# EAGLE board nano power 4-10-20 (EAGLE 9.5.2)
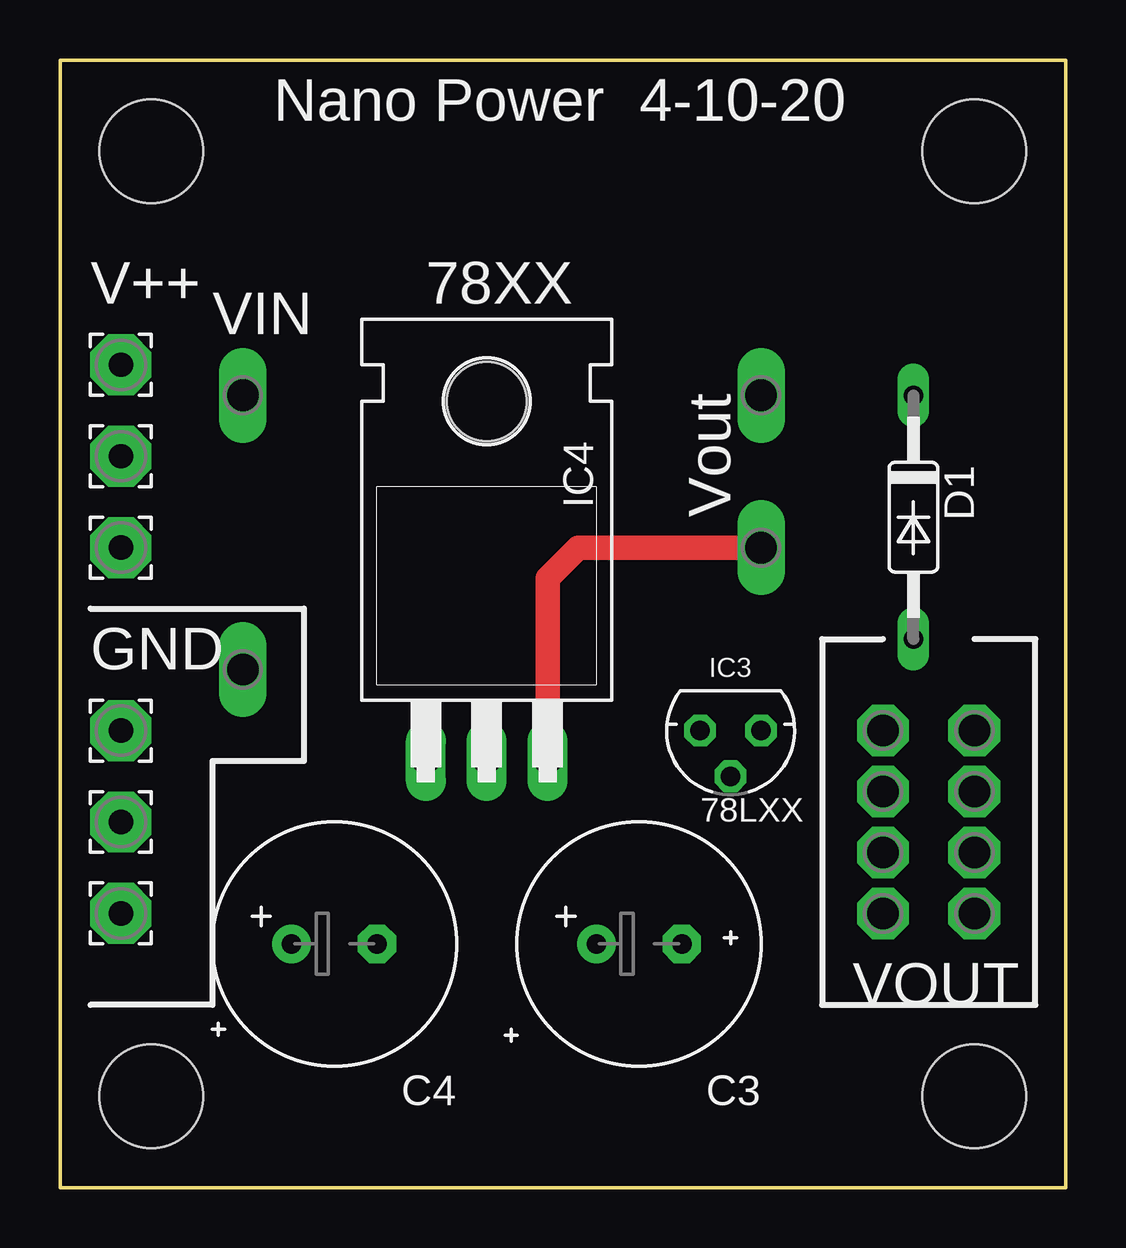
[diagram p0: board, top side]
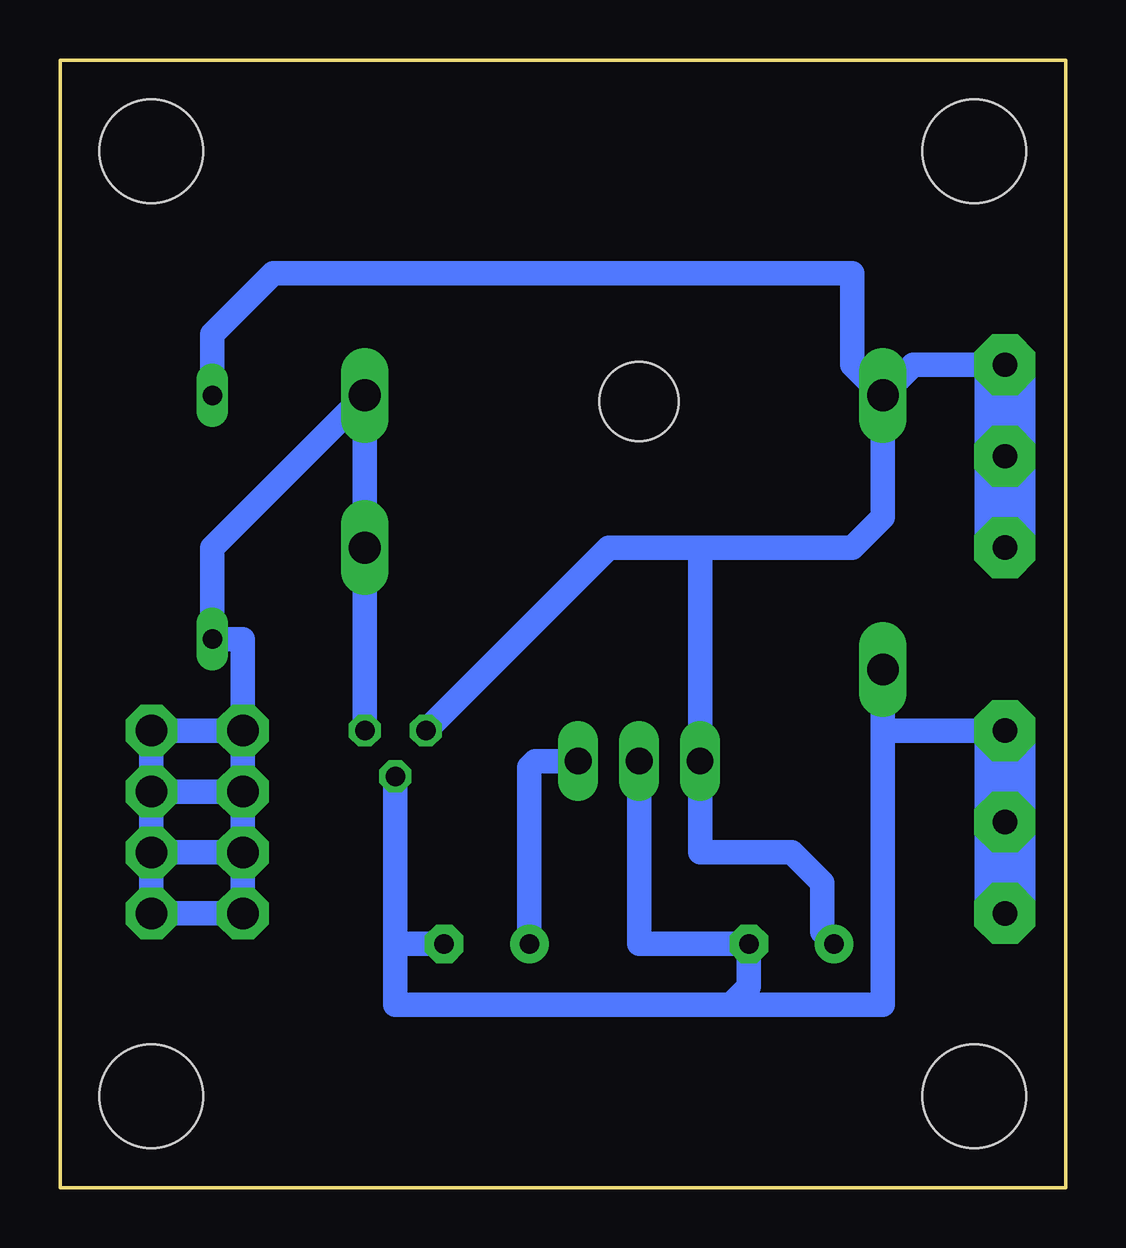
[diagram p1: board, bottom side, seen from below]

Size 41.91 x 46.99 mm. Coordinates in mm from the lower left corner, seen from the top.
Outline: 0,46.99 0,0 41.91,0 41.91,46.99 0,46.99
Copper layers (1*16): Top 0.035mm / dielectric 1.5mm / Bottom 0.035mm
Design rules "default": minimum track width 6mil, minimum drill 0.35mm, track to track 6mil, track to pad 6mil, pad to pad 6mil, via to via 6mil, smd to smd 6mil, copper to edge 40mil, drill to drill 6mil, minimum pad ring 10mil, minimum via ring 8mil, stop-mask expansion 4mil, vias tented up to drill 0mil, thermal gap 10mil
Holes 4.32 mm at 3.81,43.18 38.1,43.18 38.1,3.81 3.81,3.81

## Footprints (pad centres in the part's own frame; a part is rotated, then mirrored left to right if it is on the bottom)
2,54/1,0 = drill 1.016 pad 2.54 octagon: 1 0,0
E3,5-10 = drill 0.813 pad 1.6: + -1.778,0 | drill 0.813 pad 1.6 octagon: - 1.778,0
DO35-10 = drill 0.813 long: A 5.08,0; C -5.08,0
TO220H = drill 1.118 long: 1 -2.54,-10.16; 2 0,-10.16; 3 2.54,-10.16 | hole 3.302: 0,4.826
78LXX = drill 0.813 octagon: GND 0,1.905; IN 1.27,0; OUT -1.27,0
P1-13 = drill 1.321 pad 2.159 octagon: TP 0,0
P1-13Y = drill 1.321 pad 1.905 long: TP 0,0

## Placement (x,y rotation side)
.GND2  [2,54/1,0]  2.54,15.24 0 top
.V++1  [2,54/1,0]  2.54,30.48 0 top
C3  10uF  [E3,5-10]  24.13,10.16 0 top
C4  47uF  [E3,5-10]  11.43,10.16 0 top
D1  1N5404  [DO35-10]  35.56,27.94 270 top
GND1  [2,54/1,0]  2.54,19.05 0 top
GND.2  [2,54/1,0]  2.54,11.43 0 top
IC3  7808T  [TO220H]  17.78,27.94 0 top
IC4  [78LXX]  27.94,19.05 180 top
TP1  TPPAD1-13  [P1-13]  34.29,19.05 0 top
TP2  TPPAD1-13  [P1-13]  34.29,16.51 180 top
TP3  TPPAD1-13  [P1-13]  34.29,13.97 0 top
TP4  TPPAD1-13  [P1-13]  34.29,11.43 0 top
TP13  TPPAD1-13  [P1-13]  38.1,19.05 0 top
TP14  TPPAD1-13  [P1-13]  38.1,16.51 180 top
TP15  TPPAD1-13  [P1-13]  38.1,13.97 0 top
TP16  TPPAD1-13  [P1-13]  38.1,11.43 0 top
V++2  PTR1PAD1-13Y  [P1-13Y]  7.62,33.02 0 top
V++3  PTR1PAD1-13Y  [P1-13Y]  7.62,21.59 0 top
V++5  [2,54/1,0]  2.54,34.29 0 top
V++.1  [2,54/1,0]  2.54,26.67 0 top
VOUT1  PTR1PAD1-13Y  [P1-13Y]  29.21,33.02 0 top
VOUT.1  PTR1PAD1-13Y  [P1-13Y]  29.21,26.67 0 top

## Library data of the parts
.GND2 .V++1 GND1 GND.2 V++5 V++.1 = wirepad-NONAMES
C3 C4 = rcl; SPICEPREFIX: C
D1 = diode
IC3 = linear
IC4 = v-reg
TP1-TP4 TP13-TP16 V++2 V++3 VOUT1 VOUT.1 = testpad-CL

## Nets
GND: .GND2.1 C3.- C4.- GND1.1 GND.2.1 IC3.2 IC4.GND V++3.TP
OUT: C3.+ D1.A IC3.3 IC4.OUT TP1.TP TP2.TP TP3.TP TP4.TP TP13.TP TP14.TP TP15.TP TP16.TP VOUT1.TP VOUT.1.TP
V+: .V++1.1 C4.+ D1.C IC3.1 IC4.IN V++2.TP V++5.1 V++.1.1

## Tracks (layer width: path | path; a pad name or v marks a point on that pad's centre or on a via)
GND
  Bottom 1.016: 13.97,7.62 27.94,7.62 27.94,10.16 | 13.97,7.62 7.62,7.62 7.62,19.05 | 7.62,19.05 V++3.TP | 13.97,7.62 13.21,8.38 C4.- 17.78,10.16 IC3.2 | 27.94,10.16 IC4.GND | 7.62,19.05 GND1.1 | C3.- 27.94,10.16
  Bottom 2.54: GND1.1 .GND2.1 GND.2.1
OUT
  Top 1.016: IC3.3 20.32,25.4 21.59,26.67 VOUT.1.TP
  Bottom 1.016: TP1.TP 34.29,22.86 D1.A 35.56,26.67 VOUT1.TP VOUT.1.TP IC4.OUT | TP1.TP TP2.TP | TP2.TP TP3.TP | TP3.TP TP4.TP TP16.TP TP15.TP | TP15.TP TP14.TP | TP14.TP TP13.TP TP1.TP | TP2.TP TP14.TP | TP3.TP TP15.TP | C3.+ 22.35,17.53 22.1,17.78 IC3.3
V+
  Bottom 1.016: C4.+ 10.16,10.67 10.16,12.7 11.43,13.97 15.24,13.97 IC3.1 15.24,26.67 | V++2.TP 8.89,34.29 8.89,38.1 33.02,38.1 35.56,35.56 D1.C | V++2.TP 6.35,34.29 V++5.1 | 15.24,26.67 8.89,26.67 7.62,27.94 V++2.TP | 15.24,26.67 19.05,26.67 IC4.IN
  Bottom 2.54: V++5.1 .V++1.1 V++.1.1

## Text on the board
tNames: Nano Power | 4-10-20 | V++ | 78XX | VIN | Vout | GND | 78LXX | VOUT
tValues: AUDIODIWHY.BLOGSPOT.COM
